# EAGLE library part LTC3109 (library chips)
IC BOOST CONVERTER PMU 20QFN
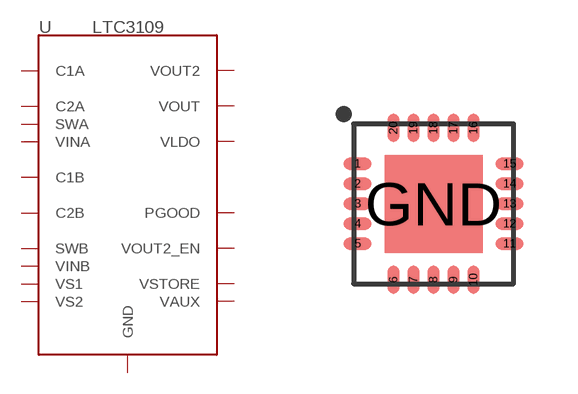
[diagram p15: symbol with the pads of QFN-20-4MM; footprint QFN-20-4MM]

Designator prefix U

## LTC3109EUF (DIGIKEY: LTC3109EUF#PBF-ND; NEWARK: 84R6674)  [QFN-20-4MM]
1  VSTORE
2  VAUX
3  VOUT
4  VOUT2
5  VOUT2_EN
6  PGOOD
7  VLDO
8  GND
9  C1B
10  C2B
11  GND
12  SWB
13  VINB
14  VINA
15  SWA
16  GND
17  C2A
18  C1A
19  VS1
20  VS2
GND  GND

## Footprint QFN-20-4MM (pad centres in mm)
smd 0.7 x 0.3: 1 -1.9,1; 2 -1.9,0.5; 3 -1.9,0; 4 -1.9,-0.5; 5 -1.9,-1; 11 1.9,-1; 12 1.9,-0.5; 13 1.9,0; 14 1.9,0.5; 15 1.9,1
smd 0.3 x 0.7: 6 -1,-1.9; 7 -0.5,-1.9; 8 0,-1.9; 9 0.5,-1.9; 10 1,-1.9; 16 1,1.9; 17 0.5,1.9; 18 0,1.9; 19 -0.5,1.9; 20 -1,1.9
smd 2.45 x 2.45: GND 0,0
